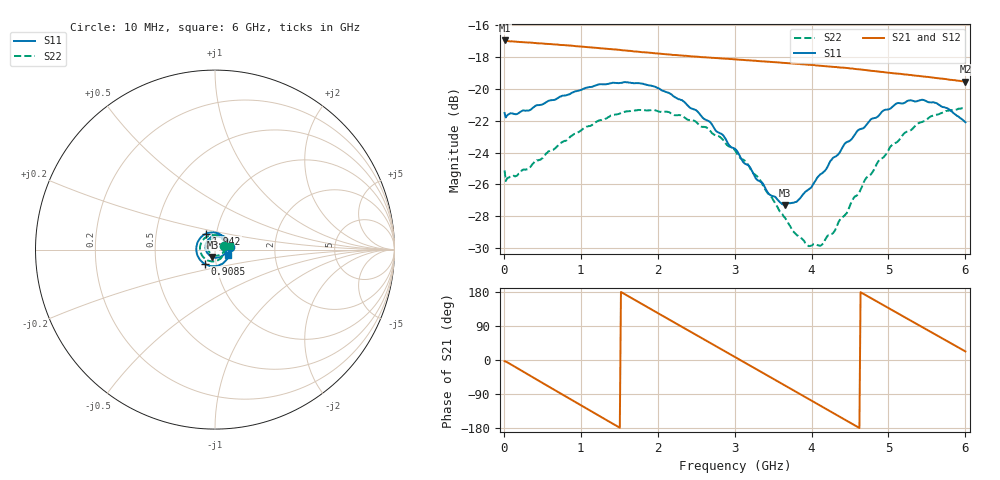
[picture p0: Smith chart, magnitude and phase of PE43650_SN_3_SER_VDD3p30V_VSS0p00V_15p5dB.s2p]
!Keysight Technologies,N5245B,MY57181451,A.13.50.07
!Date: Tuesday, May 07, 2019 08:00:16
!Correction: S11(Full 2 Port(1,2))
!S21(Full 2 Port(1,2))
!S12(Full 2 Port(1,2))
!S22(Full 2 Port(1,2))
!S2P File: Measurements: S11, S21, S12, S22:
# Hz S  dB  R 50
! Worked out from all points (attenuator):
!   401 points, 10 MHz to 6 GHz, reference 50 ohm
!   highest |S21| = -16.94 dB at 10 MHz (marker M1); lowest = -19.5 dB at 6 GHz (marker M2)
!   lowest |S11| = -27.3 dB at 3.649 GHz (marker M3), VSWR 1.09, Z = 48.4 - j3.95 ohm
!   |S11| at or under -10 dB: start of sweep to end of sweep
!   |S22| runs from -29.9 to -21.2 dB; largest |S21 - S12| = 0.0012
!   S11 on the Smith chart (normalised r, x): 10 MHz: 1.18, +0.03; 908.5 MHz: 0.88, -0.14; 1.942 GHz: 0.89, +0.16; 6 GHz: 1.15, -0.07
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1e7  -21.51 9.8  -16.94 -3.4  -16.98 -3.2  -25.12 20.5
1.74725e8  -21.57 -25.8  -17.04 -21.5  -17.08 -21.5  -25.44 -24.7
5.04175e8  -20.97 -72.3  -17.14 -60.7  -17.20 -60.7  -24.35 -71.1
9.085e8  -20.19 -124.5  -17.28 -108.6  -17.34 -108.5  -22.85 -120.2
1.013325e9  -20.04 -137.4  -17.34 -120.8  -17.38 -120.9  -22.57 -132.1
1.252925e9  -19.70 -165.1  -17.44 -149.0  -17.49 -148.9  -21.95 -157.4
1.47755e9  -19.63 169.5  -17.53 -175.2  -17.59 -175.2  -21.59 179.8
1.941775e9  -19.82 118.8  -17.74 130.8  -17.79 130.8  -21.32 134.4
2.01665e9  -19.97 110.9  -17.77 122.1  -17.83 122.1  -21.42 127.4
2.4659e9  -21.27 61.1  -17.95 70.2  -18.01 70.2  -21.98 84.1
2.750425e9  -22.59 28.7  -18.05 37.3  -18.11 37.3  -22.91 56.0
3.005e9  -23.77 -4.4  -18.13 7.9  -18.19 7.9  -23.85 29.8
3.3045e9  -25.76 -48.5  -18.24 -26.8  -18.29 -26.7  -25.56 -5.1
3.648925e9  -27.29 -109.6  -18.36 -66.6  -18.40 -66.6  -28.07 -51.7
3.7837e9  -27.12 -135.0  -18.40 -82.3  -18.45 -82.2  -29.07 -73.9
4.008325e9  -26.11 -174.4  -18.48 -108.2  -18.54 -108.2  -29.84 -116.0
4.128125e9  -25.33 167.8  -18.54 -122.1  -18.59 -122.1  -29.82 -138.8
4.277875e9  -24.34 146.3  -18.60 -139.5  -18.66 -139.4  -29.07 -165.9
4.517475e9  -23.18 115.3  -18.71 -167.2  -18.77 -167.1  -27.12 155.6
5.01165e9  -21.26 62.5  -18.98 135.8  -19.03 136.0  -23.74 97.8
5.475875e9  -20.73 19.4  -19.22 82.5  -19.27 82.7  -22.00 54.8
6e9  -22.09 -22.9  -19.53 22.7  -19.58 22.8  -21.27 12.5
